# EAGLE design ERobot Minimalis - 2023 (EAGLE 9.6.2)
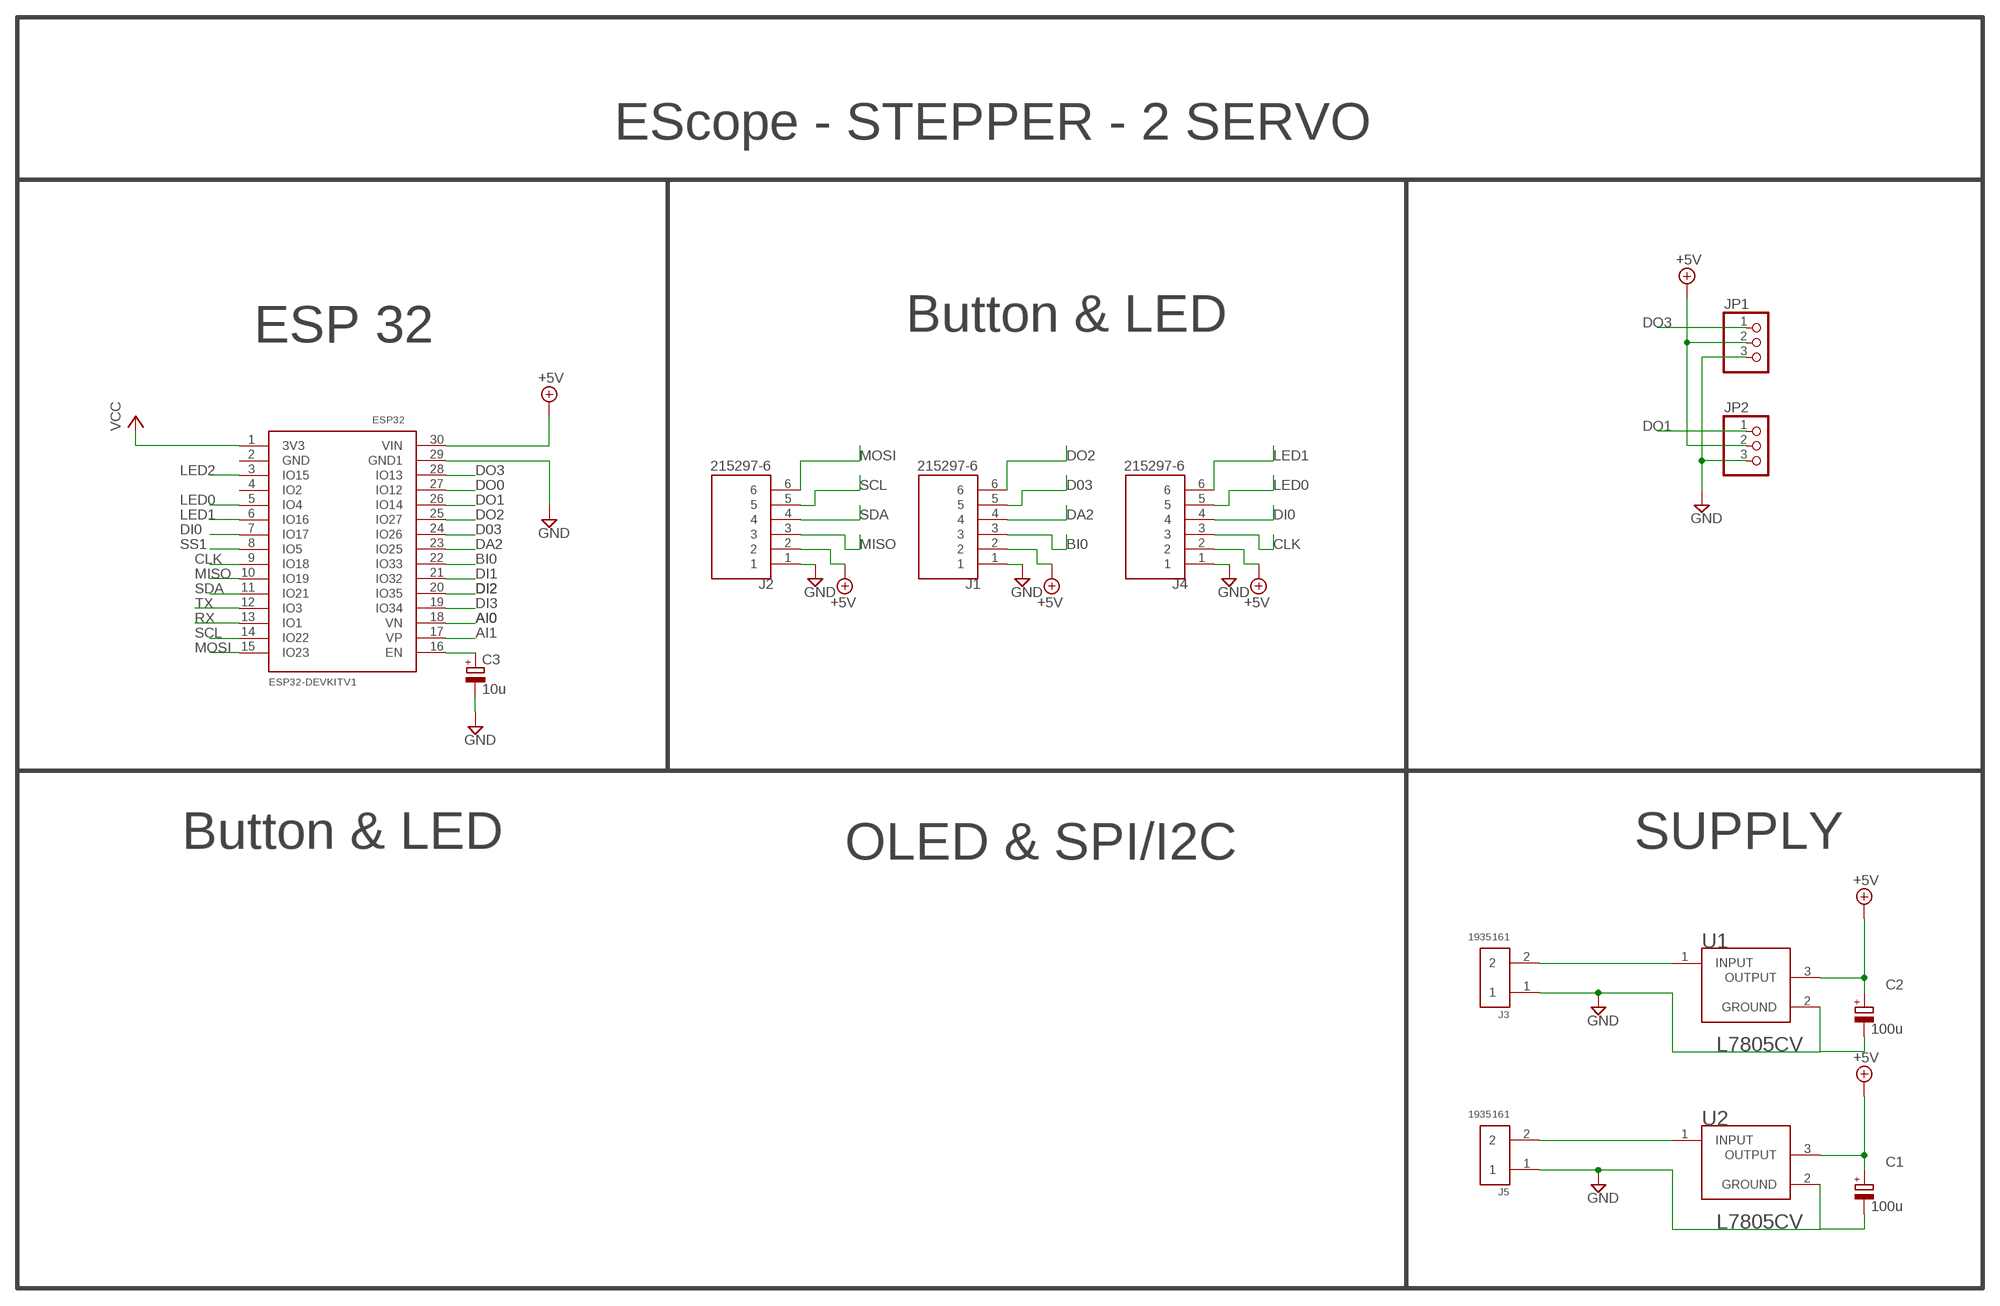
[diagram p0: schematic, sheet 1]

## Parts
C1  100u  CPOL-EUE3.5-8  [E3,5-8]
C2  100u  CPOL-EUE3.5-8  [E3,5-8]
C3  10u  CPOL-EUE2.5-5  [E2,5-5]
ESP32  DEVKIT-V1  ESP32DEVKITV1  [ESP32-DEVKITV1]
J1  215297-6  [TE_215297-6]
J2  215297-6  [TE_215297-6]
J3  1935161  [PHOENIX_1935161]
J4  215297-6  [TE_215297-6]
J5  1935161  [PHOENIX_1935161]
JP1  PINHD-1X3  [1X03]
JP2  PINHD-1X3  [1X03]
U1  STMICROELECTRONICS_L7805CVSTMICROELECTRONICS_L7805CV_0_0  [STMICROELECTRONICS_L7805CV_0]
U2  STMICROELECTRONICS_L7805CVSTMICROELECTRONICS_L7805CV_0_0  [STMICROELECTRONICS_L7805CV_0]

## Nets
+5V: C1.+ C2.+ ESP32.30(VIN) J1.2 J2.2 J4.2 JP1.2 JP2.2 U1.3(OUTPUT) U2.3(OUTPUT)
AI0: ESP32.18(VN)
AI1: ESP32.17(VP)
BI0: ESP32.22(IO33) J1.3
CLK: ESP32.9(IO18) J4.3
D03: ESP32.24(IO26) J1.5
DA2: ESP32.23(IO25) J1.4
DI0: ESP32.7(IO17) J4.4
DI1: ESP32.21(IO32)
DI2: ESP32.20(IO35)
DI3: ESP32.19(IO34)
DO0: ESP32.27(IO12)
DO1: ESP32.26(IO14) JP2.1
DO2: ESP32.25(IO27) J1.6
DO3: ESP32.28(IO13) JP1.1
GND: C1.- C2.- C3.- ESP32.29(GND1) J1.1 J2.1 J3.1 J4.1 J5.1 JP1.3 JP2.3 U1.2(GROUND) U2.2(GROUND)
LED0: ESP32.5(IO4) J4.5
LED1: ESP32.6(IO16) J4.6
LED2: ESP32.3(IO15)
MISO: ESP32.10(IO19) J2.3
MOSI: ESP32.15(IO23) J2.6
N$1: J5.2 U2.1(INPUT)
N$2: J3.2 U1.1(INPUT)
N$4: C3.+ ESP32.16(EN)
RX: ESP32.13(IO1)
SCL: ESP32.14(IO22) J2.5
SDA: ESP32.11(IO21) J2.4
SS1: ESP32.8(IO5)
TX: ESP32.12(IO3)
VCC: ESP32.1(3V3)
Unconnected: ESP32.2(GND) ESP32.4(IO2)

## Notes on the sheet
- EScope - STEPPER - 2 SERVO
- Button & LED
- ESP 32
- Button & LED | SUPPLY
- OLED & SPI/I2C

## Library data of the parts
C1-C3 = rcl:CPOL-EU: POLARIZED CAPACITOR, European symbol; SPICEPREFIX: C
ESP32 = ESP32-DEVKITV1:ESP32DEVKITV1
J1 J2 J4 = 215297-6:215297-6: Check availability; AVAILABILITY: In Stock; COMMENT: 215297-6; DESCRIPTION: Wire-To-Board Connector, Vertical, Ampmodu Hv-100 Series, Through Hole, Receptacle, 6, 2.54 Mm; EU_ROHS_COMPLIANCE: Compliant; MF: TE Connectivity; MP: 215297-6; PACKAGE: None; PRICE: None; PURCHASE-URL: https://pricing.snapeda.com/search/part/215297-6/?ref=eda
J3 J5 = 1935161:1935161: Conn Terminal Blocks 2 POS 5mm Solder ST Thru-Hole 16A Check availability; AVAILABILITY: In Stock; DESCRIPTION: 2 Position Wire to Board Terminal Block Horizontal with Board 0.197 (5.00mm) Through Hole; MF: Phoenix Contact; MP: 1935161; PACKAGE: None; PRICE: None; PURCHASE-URL: https://pricing.snapeda.com/search/part/1935161/?ref=eda
JP1 JP2 = pinhead:PINHD-1X3: PIN HEADER
U1 U2 = STMicroelectronics - L7805CV:STMICROELECTRONICS_L7805CV: Linear Voltage Regulator IC Positive Fixed 1 Output 5V 1.5A TO-220AB; CENTROID_NOT_SPECIFIED: No; DATASHEET: http://www.st.com/content/ccc/resource/technical/document/datasheet/41/4f/b3/b0/12/d4/47/88/CD00000444.pdf/files/CD00000444.pdf/jcr:content/translations/en.CD00000444.pdf; DIGIKEY_DESCRIPTION: IC REG LINEAR 5V 1.5A TO220AB; DIGIKEY_PART_NUMBER: 497-1443-5-ND; IPC_LAND_PATTERN_NAME: TO-220; LEAD_FREE: yes; MF: STMicroelectronics; MFG_PACKAGE_IDENT: TO-220-3; MOUSER_PART_NUMBER: 511-L7805CV; MPN: L7805CV; PACKAGE: TO-220-3; PREFIX: U; ROHS: yes; TEMPERATURE_RANGE_HIGH: +125°C; TEMPERATURE_RANGE_LOW: 0°C

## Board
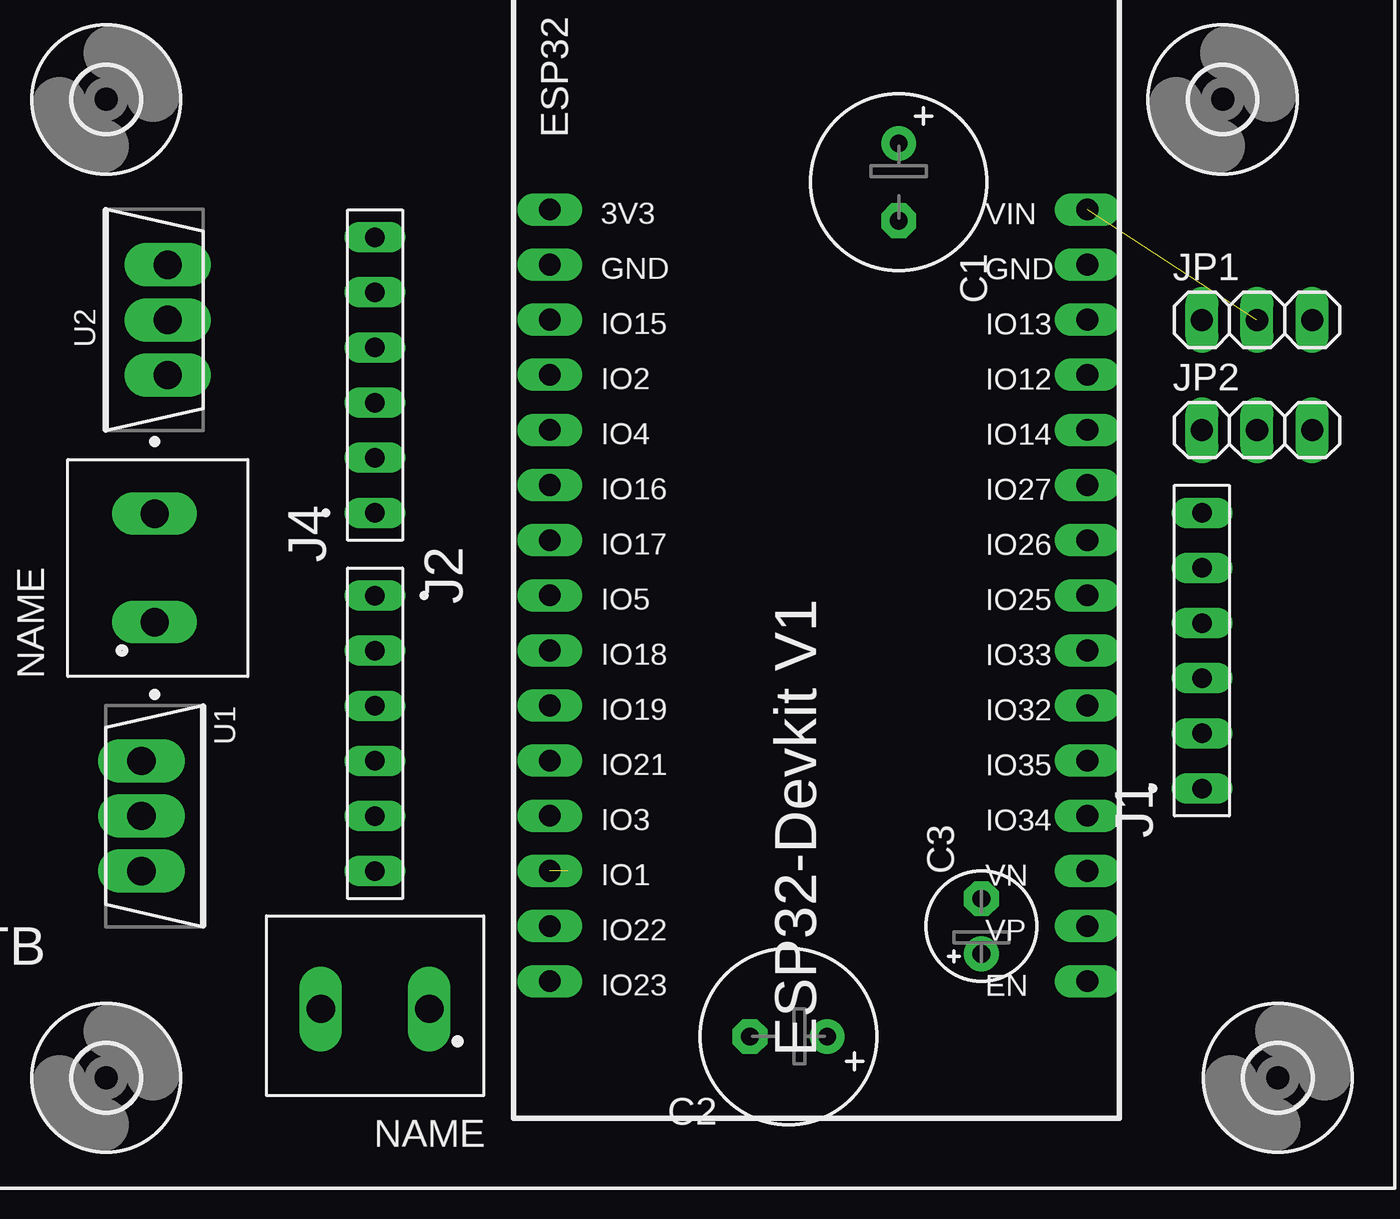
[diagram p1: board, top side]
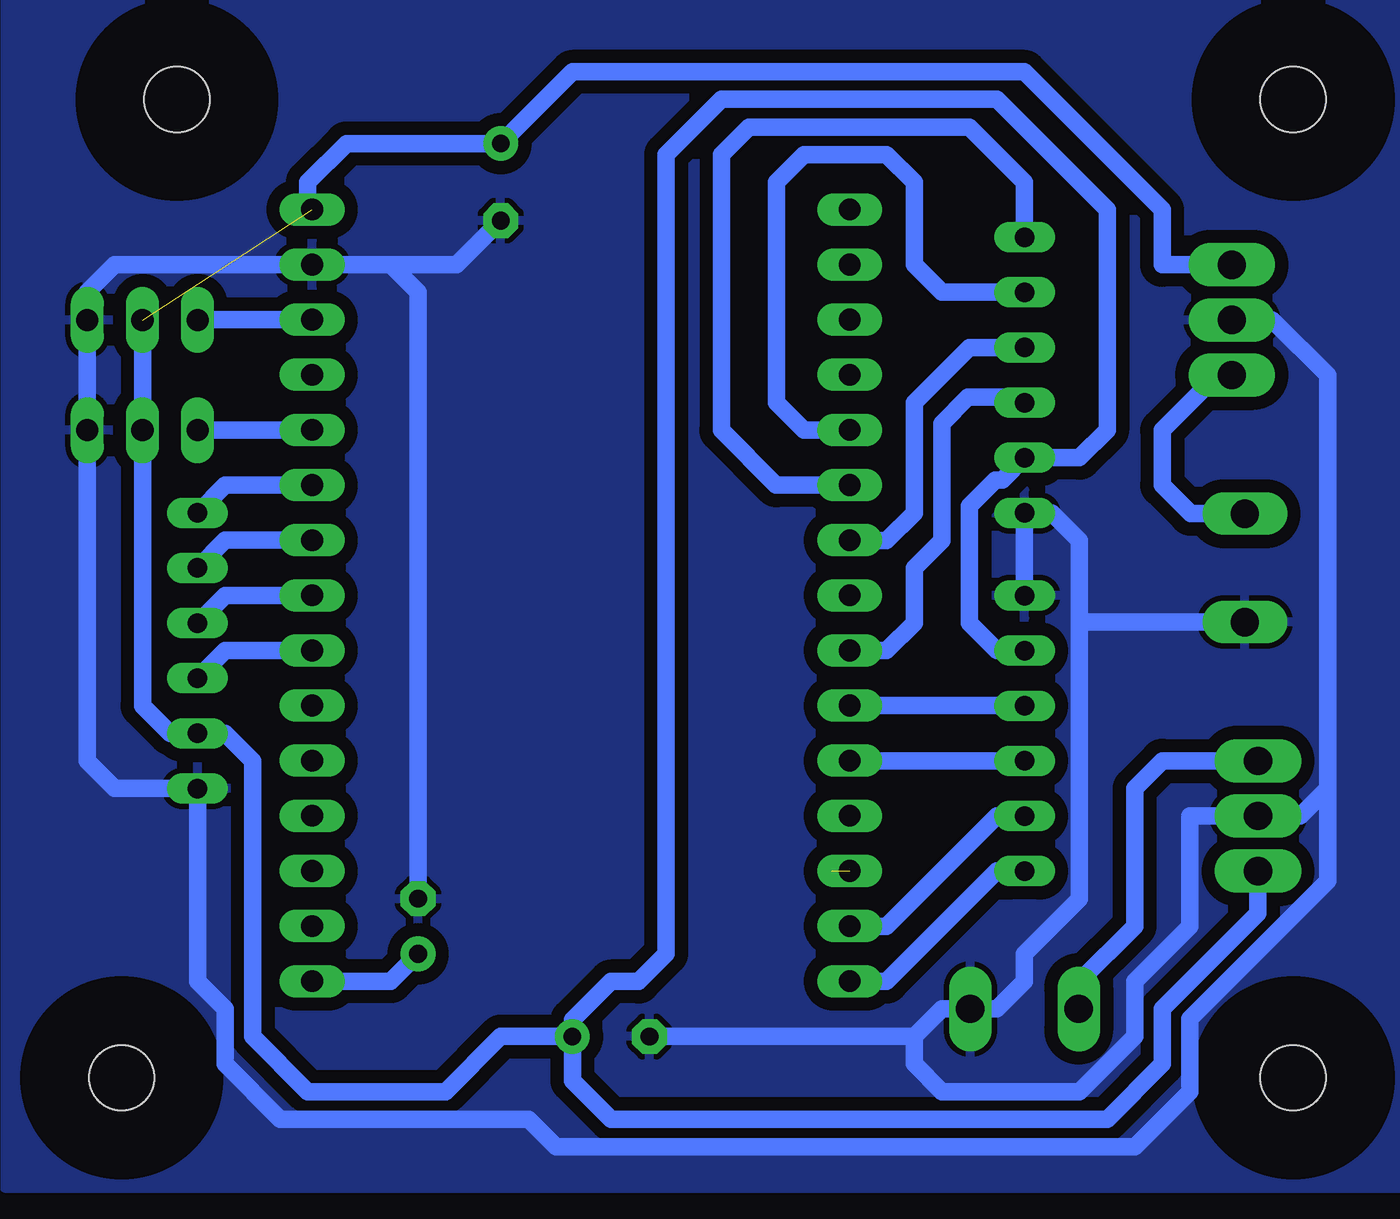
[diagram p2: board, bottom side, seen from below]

No outline drawn. Coordinates in mm, seen from the top.
Copper layers (1*16): Top 0.035mm / dielectric 1.5mm / Bottom 0.035mm
Design rules "default *": minimum track width 6mil, minimum drill 0.35mm, track to track 16mil, track to pad 16mil, pad to pad 16mil, via to via 16mil, smd to smd 16mil, copper to edge 40mil, drill to drill 6mil, minimum pad ring 10mil, minimum via ring 8mil, stop-mask expansion 4mil, vias tented up to drill 0mil, thermal gap 10mil

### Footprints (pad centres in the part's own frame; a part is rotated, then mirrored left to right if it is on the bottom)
E3,5-8 = drill 0.813 pad 1.6: + -1.778,0 | drill 0.813 pad 1.6 octagon: - 1.778,0
E2,5-5 = drill 0.813 pad 1.6: + -1.27,0 | drill 0.813 pad 1.6 octagon: - 1.27,0
ESP32-DEVKITV1 = drill 1 pad 1.422 long: 1 -22.87,-13.54; 2 -20.33,-13.54; 3 -17.79,-13.54; 4 -15.25,-13.54; 5 -12.71,-13.54; 6 -10.17,-13.54; 7 -7.63,-13.54; 8 -5.09,-13.54; 9 -2.55,-13.54; 10 -0.01,-13.54; 11 2.53,-13.54; 12 5.07,-13.54; 13 7.61,-13.54; 14 10.15,-13.54; 15 12.69,-13.54; 16 12.69,11.23; 17 10.15,11.23; 18 7.61,11.23; 19 5.07,11.23; 20 2.53,11.23; 21 -0.01,11.23; 22 -2.55,11.23; 23 -5.09,11.23; 24 -7.63,11.23; 25 -10.17,11.23; 26 -12.71,11.23; 27 -15.25,11.23; 28 -17.79,11.23; 29 -20.33,11.23; 30 -22.87,11.23
TE_215297-6 = drill 0.9 long: 1 -6.35,0; 2 -3.81,0; 3 -1.27,0; 4 1.27,0; 5 3.81,0; 6 6.35,0
PHOENIX_1935161 = drill 1.3 long: 1 -2.5,0; 2 2.5,0
1X03 = drill 1.016 long: 1 -2.54,0; 2 0,0; 3 2.54,0
STMICROELECTRONICS_L7805CV_0 = drill 1.3 pad 2 long: 1 -0.605,2.54; 2 -0.605,0; 3 -0.605,-2.54
3,0 = hole 3: 0,0

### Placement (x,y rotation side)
C1  41.91,46.99 270 top
C2  36.83,7.62 180 top
C3  45.72,12.7 90 top
ESP32  39.37,22.86 270 top
J1  55.88,25.4 90 top
J2  17.78,21.59 270 top
J3  17.78,8.89 180 top
J4  17.78,38.1 90 top
J5  7.62,29.21 90 top
JP1  58.42,40.64 0 top
JP2  58.42,35.56 0 top
U1  7.62,17.78 0 top
U2  7.62,40.64 180 top
U$2  [3,0]  56.83,50.8 0 top
U$3  [3,0]  59.37,5.71 0 top
U$4  [3,0]  5.4,5.71 0 top
U$5  [3,0]  5.4,50.8 0 top

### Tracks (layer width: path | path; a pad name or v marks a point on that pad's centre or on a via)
+5V  (1 unrouted)
  Bottom 0.813: J2.2 19.05,25.4 20.32,26.67 20.32,32.06 19.11,33.27 18.8,33.27 J4.2 15.24,34.29 13.97,35.56 13.97,45.72 19.05,50.8 31.75,50.8 34.29,48.26 34.29,11.43 35.56,10.16 36.83,10.16 38.61,8.38 C2.+ | JP1.2 JP2.2 58.42,22.86 57.15,21.59 J1.2 54.61,21.59 53.34,20.32 53.34,7.62 50.8,5.08 44.45,5.08 41.91,7.62 C2.+ | C2.+ 38.61,5.59 36.83,3.81 13.97,3.81 11.43,6.35 11.43,8.89 7.01,13.3 U1.3 | U2.3 11.43,43.18 11.43,45.72 17.78,52.07 38.61,52.07 C1.+ 49.02,48.77 50.8,46.99 50.8,45.93 ESP32.30
BI0
  Bottom 0.813: ESP32.22 54.6,25.41 J1.3
CLK
  Bottom 0.813: J4.3 18.03,37.08 20.38,37.08 21.59,35.87 21.59,30.48 22.86,29.21 22.86,26.67 24.13,25.4 ESP32.9
D03
  Bottom 0.813: ESP32.24 54.6,30.49 J1.5
DA2
  Bottom 0.813: ESP32.23 54.6,27.95 J1.4
DI0
  Bottom 0.813: J4.4 20.32,39.37 22.86,36.83 22.86,31.75 24.13,30.48 ESP32.7
DO1
  Bottom 0.813: JP2.1 ESP32.26
DO2
  Bottom 0.813: ESP32.25 54.6,33.03 J1.6
DO3
  Bottom 0.813: ESP32.28 JP1.1
GND
  Bottom 0.813: J2.1 J4.1 16.51,31.75 15.24,30.48 15.24,26.67 | 15.24,26.67 15.24,13.97 17.78,11.43 17.78,10.16 19.05,8.89 J3.1 | J3.1 21.59,8.89 22.86,7.62 | 20.32,8.85 J3.1 | 46.99,43.18 45.72,41.91 C3.- | 46.99,43.18 ESP32.29 59.69,43.18 60.96,41.91 JP1.3 JP2.3 60.96,20.32 59.69,19.05 J1.1 55.88,10.16 54.61,8.89 54.61,6.35 52.07,3.81 40.64,3.81 39.37,2.54 12.7,2.54 10.16,5.08 10.16,8.44 3.81,14.79 3.81,19.05 | C2.- 22.86,7.62 | 3.81,19.05 3.81,38.1 6.35,40.64 U2.2 | 3.81,19.05 5.08,17.78 U1.2 10.16,17.78 10.16,12.7 12.7,10.16 12.7,7.62 15.24,5.08 21.59,5.08 22.86,6.35 22.86,7.62 | C1.- 43.94,43.18 46.99,43.18 | J5.1 15.2,26.71 15.24,26.67
  pour Bottom (isolate 0.61): 0,57.15 64.77,57.15 64.77,0.64 0,0.64
LED0
  Bottom 0.813: J4.5 21.59,41.91 22.86,43.18 22.86,46.99 24.13,48.26 27.94,48.26 29.21,46.99 29.21,36.83 27.94,35.56 ESP32.5
LED1
  Bottom 0.813: ESP32.6 29.22,33.03 31.75,35.56 31.75,48.26 30.48,49.53 20.32,49.53 17.78,46.99 J4.6
MISO
  Bottom 0.813: ESP32.10 J2.3
MOSI
  Bottom 0.813: J2.6 19.05,15.24 24.13,10.16 ESP32.15
N$1
  Bottom 0.813: U2.1 8.89,38.1 11.43,35.56 11.43,33.02 10.12,31.71 J5.2
N$2
  Bottom 0.813: J3.2 15.24,8.93 15.24,10.16 12.7,12.7 12.7,19.05 11.43,20.32 U1.1
N$4
  Bottom 0.813: ESP32.16 46.98,10.17 C3.+
RX  (1 unrouted)
  Bottom 0.813: 26.67,15.24 26.66,15.25
SCL
  Bottom 0.813: ESP32.14 24.13,12.7 19.05,17.78 J2.5
SDA
  Bottom 0.813: ESP32.11 J2.4

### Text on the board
tPlace: TF ITB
